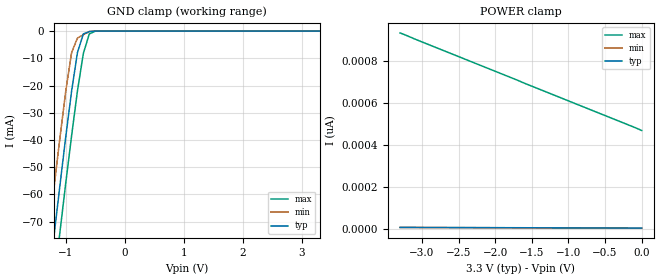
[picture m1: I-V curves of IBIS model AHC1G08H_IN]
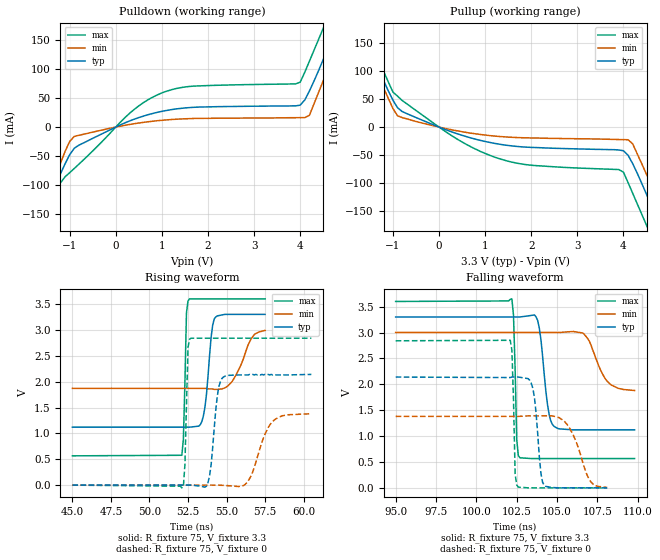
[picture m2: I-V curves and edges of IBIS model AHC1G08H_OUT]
| TEXAS INSTRUMENTS INCORPORATED
| Standard Linear and Logic Group
| IBIS Model of SN74AHC1G08H
| SINGLE 2-INPUT POSITIVE-AND GATE
| CMPAK-5 5-pin (DCK) Package
[IBIS Ver]   2.1
[Comment Char]  |_char
[File name]   ul08_3c.ibs
[File Rev]   2.0
[Date]   May 10, 2000
[Source]   Data created from SPICE simulations at Hitachi,Ltd.
[Notes]   The following is an IBIS List for the AHC1G08H.
|   Please contact sllibis@ti.com with questions and
|   comments concerning SLL IBIS models.
[Disclaimer] Property of Texas Instruments Incorporated.  Unauthorized
   reproduction and/or distribution is strictly prohibited.
   This product is protected under copyright law.
   Created 2000, (C) Copyright 2000, Texas Instruments Inc.,
   All Rights Reserved.
   UNLESS THERE IS A SIGNED, WRITTEN AGREEMENT TO THE
   CONTRARY, TEXAS INSTRUMENTS () IS PROVIDING THE IBIS
   MODELS  AND WITHOUT ANY WARRANTY, EXPRESSED OR
   IMPLIED.  TI assumes no liability for:
   1) the accuracy of the IBIS models provided to your
   company;
   2) the proper functioning of these IBIS Models in your
   design or for any resulting applications; or
   3) infringement of patents, copyrights or intellectual
   property rights resulting from your use of these IBIS
   models.
   TI provides IBIS Models as a service to our customers.
   You and your company shall not distribute, sell or give
   these models to anyone else without prior written
   permission from TI.
   TI reserves the right to make changes to our products or
   to discontinue any semiconductor product or service
   without notice, and advises our customers to obtain the
   latest version of relevant information to verify, before
   placing orders, that the information being relied on is
   current.
   Please be aware that your receipt and use of the IBIS
   information provided shall serve as acceptance of these
   terms and conditions.  If you do not accept these terms,
   you should return or destroy the IBIS models and any
   other accompanying information immediately.
|   Component AHC1G08H
[Component]   AHC1G08H
[Manufacturer]   Hitachi, Ltd.
[Package]
|   typ   min   max
R_pkg   0.090   0.051   0.105
L_pkg   1.500nH   0.940nH   1.700nH
C_pkg   0.170pF   0.110pF   0.360pF
[Pin]   signal_name   model_name   R_pin   L_pin   C_pin
1   A   AHC1G08H_IN   0.098   1.590nH   0.110pF
2   B   AHC1G08H_IN   0.051   0.940nH   0.170pF
3   GND   GND   0.092   1.590nH   0.360pF
4   Y   AHC1G08H_OUT   0.105   1.700nH   0.110pF
5   VCC   POWER   0.104   1.690nH   0.110pF
| Models and submodels in the file (2): AHC1G08H_IN (Input), AHC1G08H_OUT (Output)
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|   Model AHC1G08H_IN
[Model]   AHC1G08H_IN
Model_type  Input
Polarity   Inverting
Vinl = 0.99
Vinh = 2.31
| variable   typ   min   max
C_comp   1.80pF   1.73pF   1.97pF
[Temperature Range]   25   85   -40
[Voltage Range]   3.3   3.0   3.6
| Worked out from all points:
|   GND clamp passes 1 mA (typ) near -0.70 V on its own axis
[GND Clamp]
|   Voltage   I(typ)   I(min)   I(max)
-3.3V     -486mA     -469mA     -503mA
-1.3V     -94.6mA    -76.9mA    -112mA
-1.2V     -75.8mA    -58.1mA    -93.1mA
-1.1V     -57.3mA    -39.8mA    -74.5mA
-1V       -39.2mA    -22.4mA    -56.2mA
-900mV    -22.2mA    -7.98mA    -38.6mA
-800mV    -7.87mA    -2.53mA    -22mA
-700mV    -1.03mA    -1.34mA    -8.2mA
-600mV    -206uA     -154uA     -1.06mA
-500mV    -11.2uA    -2.6uA     -57.2uA
3.3V      3.55pA     3.3pA      469pA
[POWER Clamp]
|   Voltage   I(typ)   I(min)   I(max)
-3.3V     7pA        6.6pA      934pA
-1.6V     5.23pA     4.9pA      694pA
-100mV    3.66pA     3.4pA      484pA
0V        3.55pA     3.3pA      469pA
|   Model AHC1G08H_OUT
[Model]   AHC1G08H_OUT
Model_type  Output
Polarity   Inverting
Vmeas = 1.65
Cref = 15pf
| variable   typ   min   max
C_comp   3.84pF   3.72pF   3.96pF
[Temperature Range]   25   85   -40
[Voltage Range]   3.3   3.0   3.6
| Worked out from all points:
|   slope of the pulldown table from 0 to 0.495 V, typ, clamps not added: 30.4 ohm
|   slope of the pullup table from 0 to 0.495 V, typ, clamps not added: 34 ohm
|   rising waveform, R_fixture 75, V_fixture 3.3: 20-80 % time 383ps typ, 945ps min, 149ps max; typ from 1.12 V to 3.3 V
|   falling waveform, R_fixture 75, V_fixture 3.3: 20-80 % time 436ps typ, 915ps min, 150ps max; typ from 3.3 V to 1.12 V
|   falling waveform, R_fixture 75, V_fixture 0: 20-80 % time 344ps typ, 955ps min, 139ps max; typ from 2.14 V to 0 V
|   rising waveform, R_fixture 75, V_fixture 0: 20-80 % time 387ps typ, 967ps min, 150ps max; typ from 0 V to 2.14 V
[Pulldown]
|   Voltage   I(typ)   I(min)   I(max)
-3.3V     -489mA     -473mA     -506mA
-1.8V     -194mA     -179mA     -211mA
-1.6V     -156mA     -142mA     -173mA
-1.2V     -81mA      -62.6mA    -96.6mA
-900mV    -36.6mA    -16.1mA    -71.6mA
1V        27.2mA     11.7mA     59.1mA
3.9V      36.7mA     16.2mA     74.7mA
4.1V      47mA       16.4mA     95.1mA
4.5V      117mA      80.2mA     171mA
4.8V      174mA      137mA      229mA
5V        213mA      175mA      268mA
6.6V      528mA      491mA      584mA
[Pullup]
|   Voltage   I(typ)   I(min)   I(max)
-3.3V     491mA      474mA      508mA
-1.8V     196mA      179mA      214mA
-1.6V     157mA      141mA      175mA
-1V       47.9mA     33.1mA     62.4mA
-900mV    34.5mA     20mA       55.1mA
1.2V      -29mA      -16mA      -53.4mA
3.9V      -40.8mA    -22.2mA    -75.7mA
4.2V      -65.2mA    -30mA      -118mA
4.5V      -120mA     -84.4mA    -175mA
4.8V      -177mA     -138mA     -233mA
5V        -216mA     -177mA     -272mA
6.6V      -533mA     -494mA     -589mA
[Ramp]
| variable   typ   min   max
dV/dt_r   1.28E+00/3.80E-10   8.28E-01/9.60E-10   1.71E+00/1.50E-10
dV/dt_f   1.31E+00/4.30E-10   6.76E-01/9.40E-10   1.82E+00/1.40E-10
R_load = 75
[Rising Waveform]
R_fixture = 75
V_fixture = 3.3
V_fixture_min = 3.0
V_fixture_max = 3.6
|   Time   V(typ)   V(min)   V(max)
45ns      1.12V      1.87V      566mV
52.1ns    1.12V      1.87V      577mV
52.2ns    1.12V      1.87V      883mV
52.4ns    1.12V      1.87V      3.33V
52.5ns    1.12V      1.87V      3.56V
53.5ns    1.34V      1.87V      3.6V
54.2ns    3.21V      1.85V      3.6V
55.3ns    3.3V       1.98V      3.6V
56.6ns    3.3V       2.83V      3.6V
57.5ns    3.3V       2.99V      3.6V
[Falling Waveform]
R_fixture = 75
V_fixture = 3.3
V_fixture_min = 3.0
V_fixture_max = 3.6
|   Time   V(typ)   V(min)   V(max)
95ns      3.3V       3V         3.6V
102.2ns   3.3V       3V         3.65V
102.3ns   3.3V       3V         3.33V
102.5ns   3.3V       3V         932mV
102.6ns   3.3V       3V         620mV
103.8ns   3.23V      3V         566mV
104.8ns   1.19V      3V         566mV
106.6ns   1.12V      2.99V      566mV
108.1ns   1.12V      2.06V      566mV
109.8ns   1.12V      1.88V      566mV
[Falling Waveform]
R_fixture = 75
V_fixture = 0
|   Time   V(typ)   V(min)   V(max)
95ns      2.14V      1.38V      2.84V
102.1ns   2.13V      1.38V      2.85V
102.2ns   2.14V      1.38V      2.66V
102.4ns   2.14V      1.38V      268mV
102.5ns   2.14V      1.38V      54.3mV
103.5ns   1.92V      1.39V      79uV
104.2ns   48mV       1.39V      -70uV
105.5ns   118uV      1.27V      48uV
107ns     39uV       159mV      -28uV
108.1ns   -19uV      8.63mV     18uV
[Rising Waveform]
R_fixture = 75
V_fixture = 0
|   Time   V(typ)   V(min)   V(max)
45ns      0V         0V         0V
52.2ns    51uV       -16uV      -28.6mV
52.3ns    337uV      -17uV      395mV
52.5ns    824uV      -19uV      2.66V
52.7ns    829uV      -21uV      2.84V
53.8ns    52.7mV     599uV      2.84V
54.8ns    2.09V      -4.64mV    2.84V
56.4ns    2.13V      80.6mV     2.84V
58.1ns    2.14V      1.26V      2.84V
60.5ns    2.14V      1.38V      2.84V
